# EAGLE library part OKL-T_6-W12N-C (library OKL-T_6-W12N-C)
Non-Isolated PoL Module DC DC Converter 1 Output 0.591 ~ 5.5V 6A 4.5V - 14V Input Source: Datasheet
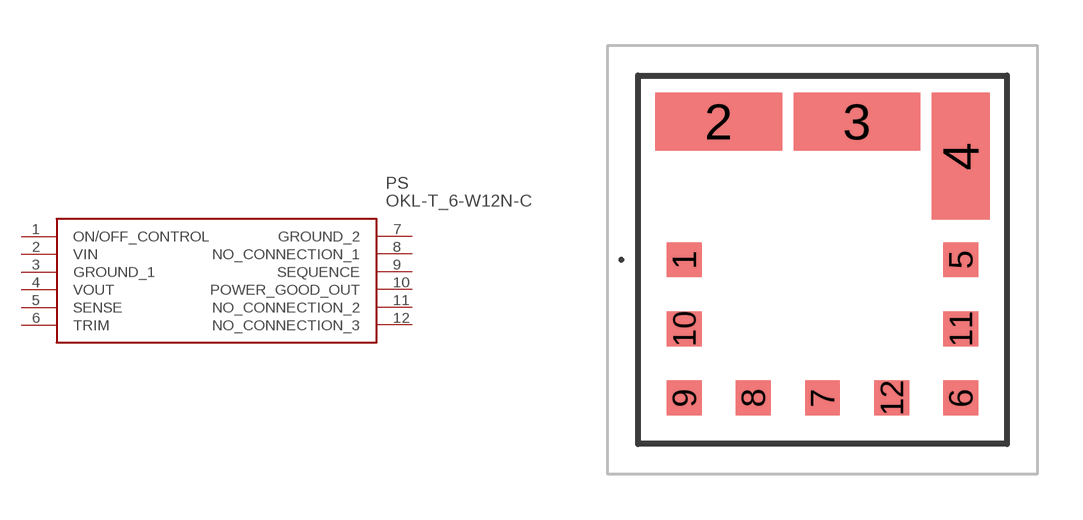
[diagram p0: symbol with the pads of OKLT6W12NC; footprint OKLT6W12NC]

Designator prefix PS

## OKL-T_6-W12N-C (Description: Non-Isolated PoL Module DC DC Converter 1 Output 0.591 ~ 5.5V 6A 4.5V - 14V Input; Height: 7.2mm; Manufacturer_Name: Murata Electronics; Manufacturer_Part_Number: OKL-T/6-W12N-C; Mouser_Part_Number: 580-OKL-T/6-W12N-C; Mouser_Price-Stock: https://www.mouser.co.uk/ProductDetail/Murata-Power-Solutions/OKL-T-6-W12N-C?qs=b1CvEdhOXIYZVD7gV2R3gw%3D%3D)  [OKLT6W12NC]
1  ON/OFF_CONTROL
2  VIN
3  GROUND_1
4  VOUT
5  SENSE
6  TRIM
7  GROUND_2
8  NO_CONNECTION_1
9  SEQUENCE
10  POWER_GOOD_OUT
11  NO_CONNECTION_2
12  NO_CONNECTION_3

## Footprint OKLT6W12NC (pad centres in mm)
OKL-T/6-W12N-C-1_2024
smd 1.145 x 1.145: 1 -4.57,0; 5 4.57,0; 6 4.57,-4.57; 7 0,-4.57; 8 -2.29,-4.57; 9 -4.57,-4.57; 10 -4.57,-2.29; 11 4.57,-2.29; 12 2.29,-4.57
smd 4.19 x 1.905: 2 -3.43,4.57; 3 1.14,4.57
smd 1.905 x 4.19: 4 4.57,3.43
